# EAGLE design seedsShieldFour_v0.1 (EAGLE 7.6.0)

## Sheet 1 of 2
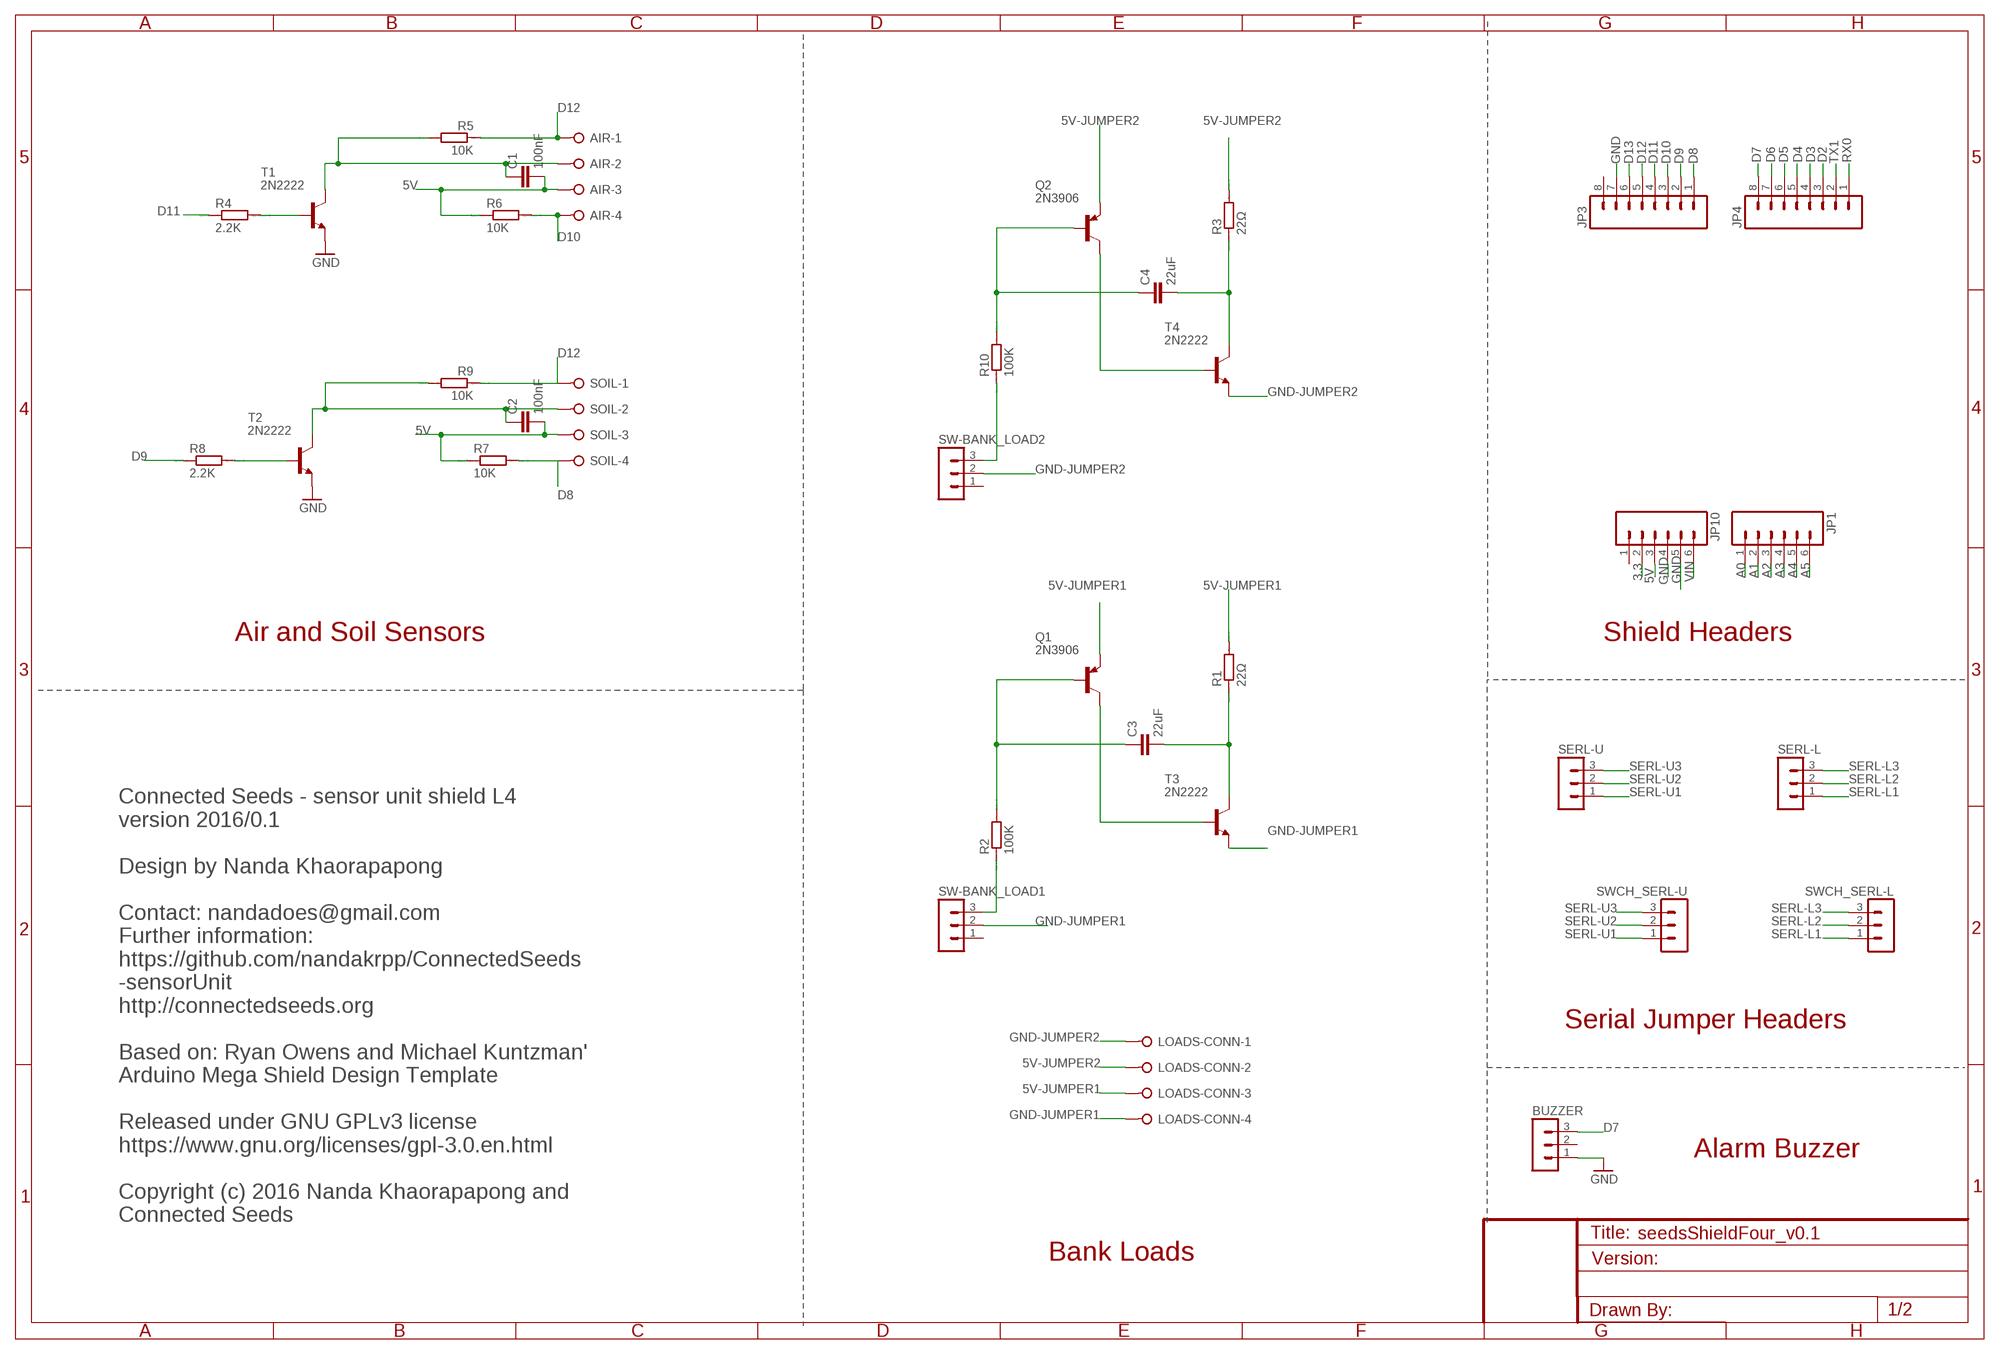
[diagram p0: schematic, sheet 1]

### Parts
AIR  W237-04P  [W237-4P]
BUZZER  MA03-1  [MA03-1]
C1  100nF  C2.5/2  [C2.5-2]
C2  100nF  C2.5/2  [C2.5-2]
C3  22uF  CAPPTH1  [CAP-PTH-5MM]
C4  22uF  CAPPTH1  [CAP-PTH-5MM]
JP1  M06LOCK  [1X06_LOCK]
JP3  M08LOCK  [1X08_LOCK]
JP4  M08LOCK  [1X08_LOCK]
JP10  M06LOCK  [1X06_LOCK]
LOADS-CONN  W237-04P  [W237-4P]
Q1  2N3906  [TO92]
Q2  2N3906  [TO92]
R1  22Ω  R0204/7  [0204/7]
R2  100K  R0204/7  [0204/7]
R3  22Ω  R0204/7  [0204/7]
R4  2.2K  R0204/7  [0204/7]
R5  10K  R0204/7  [0204/7]
R6  10K  R0204/7  [0204/7]
R7  10K  R0204/7  [0204/7]
R8  2.2K  R0204/7  [0204/7]
R9  10K  R0204/7  [0204/7]
R10  100K  R0204/7  [0204/7]
SERL-L  MA03-1  [MA03-1]
SERL-U  MA03-1  [MA03-1]
SOIL  W237-04P  [W237-4P]
SW-BANK_LOAD1  MA03-1  [MA03-1]
SW-BANK_LOAD2  MA03-1  [MA03-1]
SWCH_SERL-L  MA03-1  [MA03-1]
SWCH_SERL-U  MA03-1  [MA03-1]
T1  2N2222  [TO18]
T2  2N2222  [TO18]
T3  2N2222  [TO18]
T4  2N2222  [TO18]

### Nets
3.3: JP10.2
5V: AIR.3 C1.2 C2.2 JP10.3 R6.1 R7.1 SOIL.3
5V-JUMPER1: LOADS-CONN.3 Q1.3(E) R1.2
5V-JUMPER2: LOADS-CONN.2 Q2.3(E) R3.2
A0: JP1.1
A1: JP1.2
A2: JP1.3
A3: JP1.4
A4: JP1.5
A5: JP1.6
D2: JP4.3
D3: JP4.4
D4: JP4.5
D5: JP4.6
D6: JP4.7
D7: BUZZER.3 JP4.8
D8: JP3.1 R7.2 SOIL.4
D9: JP3.2 R8.1
D10: AIR.4 JP3.3 R6.2
D11: JP3.4 R4.1
D12: AIR.1 JP3.5 R5.1 R9.1 SOIL.1
D13: JP3.6
GND: BUZZER.1 JP3.7 JP10.4 JP10.5 T1.1(E) T2.1(E)
GND-JUMPER1: LOADS-CONN.4 SW-BANK_LOAD1.2 T3.1(E)
GND-JUMPER2: LOADS-CONN.1 SW-BANK_LOAD2.2 T4.1(E)
N$1: R8.2 T2.2(B)
N$2: C2.1 R9.2 SOIL.2 T2.3(C)
N$3: R4.2 T1.2(B)
N$4: AIR.2 C1.1 R5.2 T1.3(C)
N$5: C3.2 R1.1 T3.3(C)
N$6: C3.1 Q1.2(B) R2.2
N$7: R2.1 SW-BANK_LOAD1.3
N$8: Q1.1(C) T3.2(B)
N$9: C4.2 R3.1 T4.3(C)
N$10: C4.1 Q2.2(B) R10.2
N$11: R10.1 SW-BANK_LOAD2.3
N$12: Q2.1(C) T4.2(B)
RX0: JP4.1
SERL-L1: SERL-L.1 SWCH_SERL-L.1
SERL-L2: SERL-L.2 SWCH_SERL-L.2
SERL-L3: SERL-L.3 SWCH_SERL-L.3
SERL-U1: SERL-U.1 SWCH_SERL-U.1
SERL-U2: SERL-U.2 SWCH_SERL-U.2
SERL-U3: SERL-U.3 SWCH_SERL-U.3
TX1: JP4.2
VIN: JP10.6
Unconnected: BUZZER.2 JP3.8 JP10.1 SW-BANK_LOAD1.1 SW-BANK_LOAD2.1

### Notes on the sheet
- Air and Soil Sensors | Shield Headers
- Serial Jumper Headers
- Alarm Buzzer
- Connected Seeds - sensor unit shield L4 
  version 2016/0.1                                                                                                        
  
  Design by Nanda Khaorapapong                     
  
  Contact: nandadoes@gmail.com
  Further information:
  https://github.com/nandakrpp/ConnectedSeeds
  -sensorUnit
  http://connectedseeds.org
  
  Based on: Ryan Owens and Michael Kuntzman' 
  Arduino Mega Shield Design Template
  
  Released under GNU GPLv3 license
  https://www.gnu.org/licenses/gpl-3.0.en.html
  
  Copyright (c) 2016 Nanda Khaorapapong and 
  Connected Seeds
- Bank Loads

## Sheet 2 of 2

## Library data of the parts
AIR LOADS-CONN SOIL = con-wago-508:W237-04P: WAGO SREW CLAMP; OC_FARNELL: unknown; OC_NEWARK: unknown
BUZZER SERL-L SERL-U SW-BANK_LOAD1 SW-BANK_LOAD2 SWCH_SERL-L SWCH_SERL-U = con-lstb:MA03-1: PIN HEADER; OC_FARNELL: unknown; OC_NEWARK: unknown
C1 C2 = capacitor-wima:C: CAPACITOR
C3 C4 = SparkFun-Capacitors:CAP: Capacitor
JP1 JP10 = SparkFun:M06: Header 6 Standard 6-pin 0.1" header. Use with straight break away headers (SKU : PRT-00116), right angle break away headers (PRT-00553), swiss pins (PRT-00743), machine pins (PRT-00117), and female headers (PRT-00115). Molex polarized connector foot print use with SKU : PRT-08094 with associated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
JP3 JP4 = SparkFun:M08: Header 8 Standard 8-pin 0.1" header. Use with straight break away headers (SKU : PRT-00116), right angle break away headers (PRT-00553), swiss pins (PRT-00743), machine pins (PRT-00117), and female headers (PRT-00115).
Q1 Q2 = transistor-pnp:2N3906: PNP Transistor
R1-R10 = eagle-ltspice:R: RESISTOR, European symbol; SPICEMODEL: NONE; SPICEPREFIX: R
T1-T4 = transistor:2N2222: NPN TRANSISTOR

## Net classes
0 default: width 0.61 mm

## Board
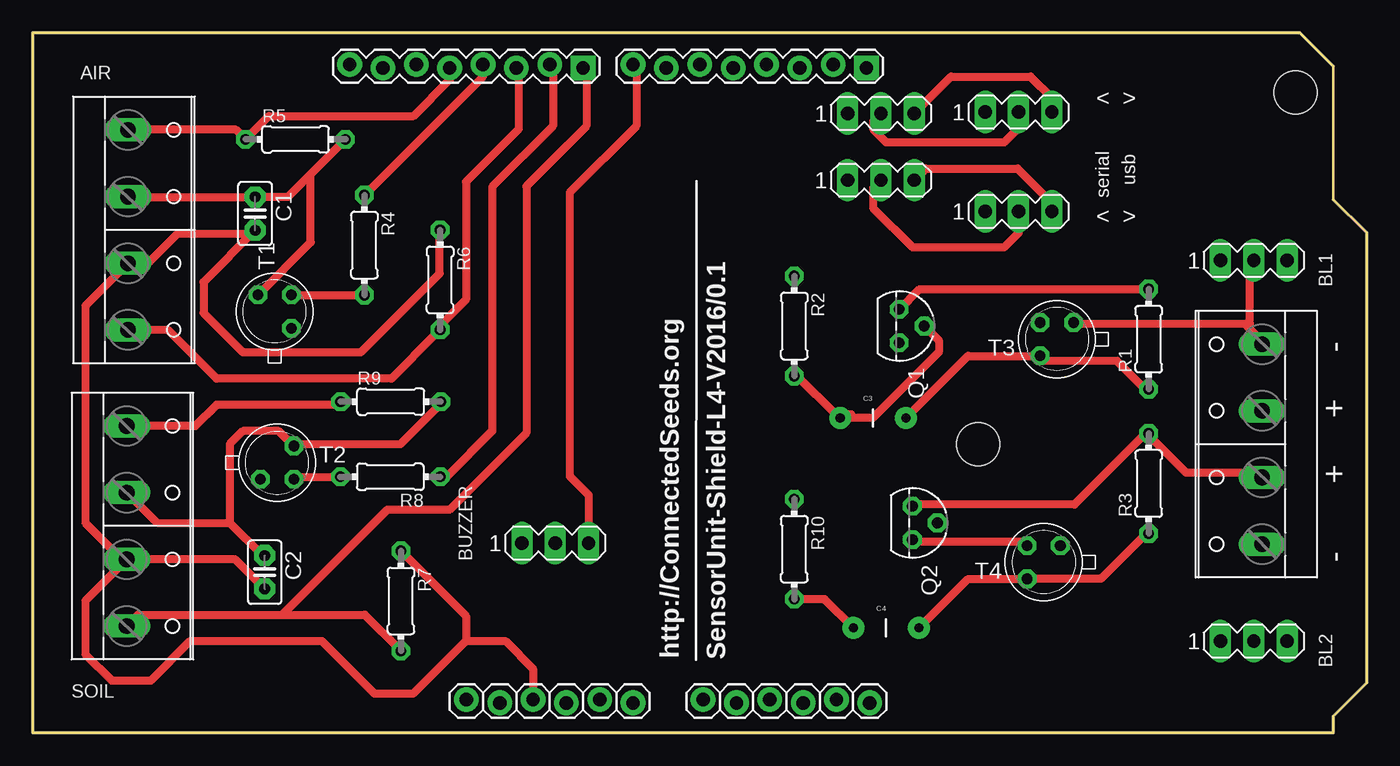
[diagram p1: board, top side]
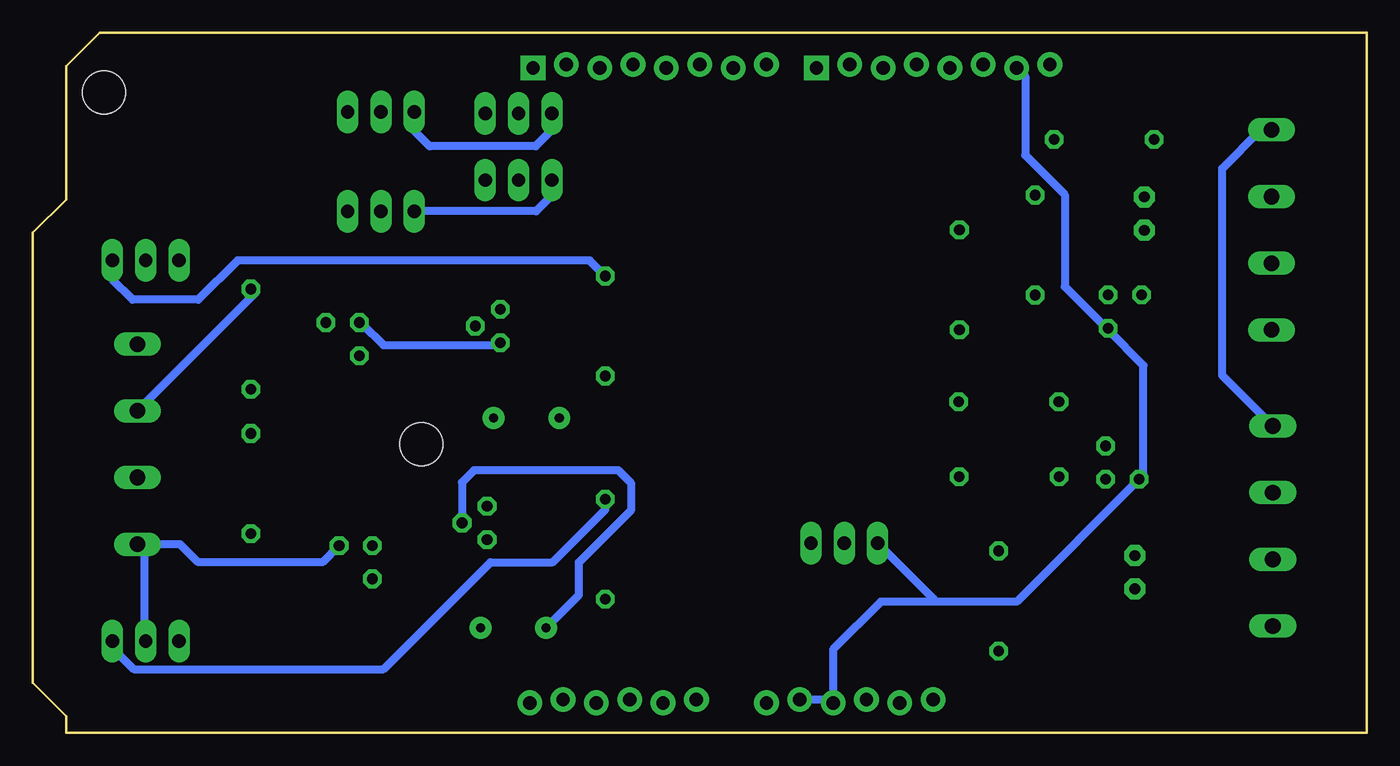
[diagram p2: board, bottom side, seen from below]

Size 101.6 x 53.34 mm. Coordinates in mm from the lower left corner, seen from the top.
Outline: 0,0 99.06,0 99.06,1.27 101.6,3.81 101.6,38.1 99.06,40.64 99.06,50.8 96.52,53.34 0,53.34 0,0
Copper layers (1*16): Top 0.035mm / dielectric 1.5mm / Bottom 0.035mm
Design rules "PCB_TRAIN *": minimum track width 0.2mm, minimum drill 0.5mm, track to track 0.2mm, track to pad 0.2mm, pad to pad 0.2mm, via to via 0.2mm, smd to smd 0.2mm, copper to edge 0.2mm, drill to drill 0.5mm, minimum pad ring 12mil, minimum via ring 10mil, stop-mask expansion 4mil, vias tented up to drill 25mil, thermal gap 10mil

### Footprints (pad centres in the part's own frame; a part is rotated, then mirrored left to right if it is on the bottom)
W237-4P = drill 1.194 long: 1 -7.62,-0.635; 2 -2.54,-0.635; 3 2.54,-0.635; 4 7.62,-0.635
MA03-1 = drill 1.016 long: 1 -2.54,0; 2 0,0; 3 2.54,0
C2.5-2 = drill 0.813 pad 1.6 octagon: 1 -1.27,0; 2 1.27,0
CAP-PTH-5MM = drill 0.7 pad 1.651: 1 -2.5,0; 2 2.5,0
1X06_LOCK = drill 1.016 pad 1.88: 1 0,0; 2 2.54,-0.254; 3 5.08,0; 4 7.62,-0.254; 5 10.16,0; 6 12.7,-0.254
1X08_LOCK = drill 1.016 pad 1.88 square: 1 0,0.127 | drill 1.016 pad 1.88: 2 2.54,-0.127; 3 5.08,0.127; 4 7.62,-0.127; 5 10.16,0.127; 6 12.7,-0.127; 7 15.24,0.127; 8 17.78,-0.127
TO92 = drill 0.813 octagon: 1 1.27,0; 2 0,1.905; 3 -1.27,0
0204/7 = drill 0.813 octagon: 1 -3.81,0; 2 3.81,0
TO18 = drill 0.813 octagon: 1 -1.27,-1.27; 2 1.27,-1.27; 3 1.27,1.27
STAND-OFF = hole 3.302: 0,0

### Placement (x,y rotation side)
AIR  7.89,38.32 270 top
BUZZER  39.79,14.46 0 top
C1  16.93,39.56 270 top
C2  17.66,12.24 270 top
C3  64,24 0 top
C4  65,8 0 top
JP1  51.05,2.54 0 top
JP3  41.91,50.8 180 top
JP4  63.5,50.8 180 top
JP10  33.02,2.54 0 top
LOADS-CONN  93,22 90 top
Q1  66,31 270 top
Q2  67,16 270 top
R1  85,30 90 top
R2  58,31 270 top
R3  85,19 90 top
R4  25.26,37.16 270 top
R5  20.01,45.23 0 top
R6  31.02,34.51 270 top
R7  28.04,10.05 270 top
R8  27.23,19.51 180 top
R9  27.26,25.24 0 top
R10  58,14 270 top
SERL-L  64.6,42.12 0 top
SERL-U  64.6,47.2 0 top
SOIL  7.79,15.76 270 top
SW-BANK_LOAD1  93,36 0 top
SW-BANK_LOAD2  93,7 0 top
SWCH_SERL-L  75.08,39.74 0 top
SWCH_SERL-U  75.08,47.3 0 top
T1  18.42,32.1 90 top
T2  18.61,20.59 0 top
T3  78,30 180 top
T4  77,13 180 top
U$4  [STAND-OFF]  96.17,48.8 0 top
U$5  [STAND-OFF]  72,22 0 top

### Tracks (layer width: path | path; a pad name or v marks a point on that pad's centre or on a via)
5V
  Top 0.61: SOIL.3 6.78,13.22 4,16 4,32.53 AIR.3 8.78,35.78 11,38 16.64,38 C1.2 13,34.36 13,32 16,29 25,29 31,35 31,38 31.02,38.02 R6.1 | SOIL.3 4,10.07 4,6 6,4 9,4 12,7 22,7 26,3 29,3 33,7 | 33,7 36,7 38.1,4.9 JP10.3 | C2.2 15.41,13.22 SOIL.3 | R7.1 33,8.9 33,7
5V-JUMPER1  (1 unrouted)
  Top 0.61: 84.6,33.6 R1.2 67.54,33.81 Q1.3
  Bottom 0.61: 84.6,33.6 93.51,24.69 LOADS-CONN.3
5V-JUMPER2
  Top 0.61: Q2.3 67.2,17.41 79.34,17.41 84.6,22.67 R3.2 85.01,22.67 87.84,19.84 93.51,19.84 LOADS-CONN.2
D7
  Top 0.61: JP4.8 45.97,50.67 45.97,46.23 40.89,41.15 40.89,19.56 42.33,18.12 BUZZER.3
D8
  Top 0.203: JP3.1 41.91,50.8
  Top 0.61: SOIL.4 8.01,9 19,9 | 19,9 25.28,9 R7.2 | JP3.1 42.16,50.42 42.16,46.23 37.59,41.66 37.59,22.86 31.73,17 27,17 19,9
D9
  Top 0.203: JP3.2 39.37,50.8
  Top 0.61: R8.1 31.51,19.51 35,23 35,41.6 39.62,46.23 39.62,50.55 39.37,50.8
D10
  Top 0.203: JP3.3 36.83,50.8
  Top 0.61: R6.2 30.66,30.34 | 30.66,30.34 27.32,27 14,27 10.3,30.7 AIR.4 | JP3.3 37,50.5 37,46 33,42 33,33 30.66,30.66 30.66,30.34
D11
  Top 0.203: JP3.4 34.29,50.8
  Top 0.61: R4.1 34.29,50 JP3.4
D12
  Top 0.203: JP3.5 31.75,50.8
  Top 0.61: JP3.5 31.75,49.75 29,47 17.97,47 R5.1 15.48,45.94 AIR.1 | R9.1 23.21,25 14,25 12.38,23.38 SOIL.1
  Bottom 0.61: SOIL.1 11,27.23 11,43 8.06,45.94 AIR.1
GND
  Bottom 0.61: 33,10 26.66,10 T2.1 17,19.66 17,28 19.69,30.69 T1.1 19.83,30.83 23,34 23,41 26,44 26,50 JP3.7 | 33,10 37,10 40.64,6.36 JP10.4 40.89,2.54 JP10.5 | BUZZER.1 33,10.21 33,10
GND-JUMPER1
  Top 0.61: 92.5,30.97 93.51,29.95 LOADS-CONN.4 | 92.5,30.97 92.29,31.17 79.34,31.17 T3.1 | SW-BANK_LOAD1.2 92.7,35.62 92.7,31.17 92.5,30.97
GND-JUMPER2
  Bottom 0.61: 93.1,13.76 93.51,14.17 LOADS-CONN.1 | 93.1,13.76 93.1,7.29 SW-BANK_LOAD2.2 | 93.1,13.76 LOADS-CONN.1 | T4.1 79.54,13 89,13 90.38,14.38 LOADS-CONN.1
N$1
  Top 0.61: T2.2 20.07,19.51 R8.2
N$2
  Top 0.61: SOIL.2 9.46,16 15,16 | 15,16 17.49,13.51 C2.1 | 15,16 15,22 16,23 18.74,23 T2.3 20.02,22 28,22 31.07,25.07 31.17,25.1 R9.2
N$3
  Top 0.61: T1.2 19.71,33.35 R4.2
N$4
  Top 0.61: AIR.2 7.29,40.83 C1.1 19.42,40.83 21.17,42.58 | R5.2 21.17,42.58 | T1.3 21.17,37.39 21.17,42.58
N$5
  Top 0.61: T3.3 76.91,28.34 82.58,28.34 84.6,26.31 R1.1 | C3.2 66.79,24.29 71.23,28.73 T3.3 | 76.51,28.34 T3.3
N$6
  Top 0.61: R2.2 58.29,27.12 61.12,24.29 C3.1 61.53,24.29 62,24.29 | 62,24.29 62.34,24.29 | Q1.2 69,29.91 69,29 64,24 62,24 62,24.29
N$7
  Bottom 0.61: R2.1 59.19,36 86,36 89,33 94,33 95.54,34.54 SW-BANK_LOAD1.3
N$8
  Bottom 0.61: Q1.1 66.39,29.55 74.89,29.55 76.51,31.17 T3.2
N$9
  Top 0.61: R3.1 84.6,14.98 81.36,11.74 76.1,11.74 T4.3 71.23,11.73 C4.2
N$10
  Top 0.61: C4.1 60.31,10.19 R10.2
  Bottom 0.61: C4.1 60,10.5 60,13 56,17 56,19 57,20 68,20 68.91,19.09 Q2.2
N$11
  Bottom 0.61: SW-BANK_LOAD2.3 95.94,6.88 93.91,4.86 74.89,4.86 66.75,13 62,13 58,17 R10.1
N$12
  Top 0.61: T4.2 75.7,14.57 67.2,14.57 Q2.1
SERL-L1
  Bottom 0.61: SERL-L.1 62,42.06 62,41 63.26,39.74 SWCH_SERL-L.1
SERL-L2
  Top 0.61: SERL-L.2 64,41.52 64,40 67,37 74,37 75.08,38.08 SWCH_SERL-L.2
SERL-L3
  Top 0.61: SERL-L.3 68.02,43 75,43 78,40 78,39 77.62,39.38 SWCH_SERL-L.3
SERL-U1
  Bottom 0.61: SERL-U.1 62,47.14 62,46 63.3,44.7 71.37,44.7 72.54,45.87 SWCH_SERL-U.1
SERL-U2
  Top 0.61: SERL-U.2 64,46.6 64,46 65,45 74,45 75.08,46.08 SWCH_SERL-U.2
SERL-U3
  Top 0.61: SERL-U.3 69.94,50 76,50 77.62,48.38 SWCH_SERL-U.3

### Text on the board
tPlace: < | > | usb | serial | < | > | http://ConnectedSeeds.org | SensorUnit-Shield-L4-V2016/0.1
tNames: BL1 | - | + | + | - | BL2
tValues: <-serial | usb->
bDocu: 9 | 8 | 7 | 12 | 11 | 10 | GND | 5V | GND | GND

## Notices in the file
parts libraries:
SparkFun-Capacitors: Licensing: Creative Commons ShareAlike 4.0 International - https://creativecommons.org/licenses/by-sa/4.0
